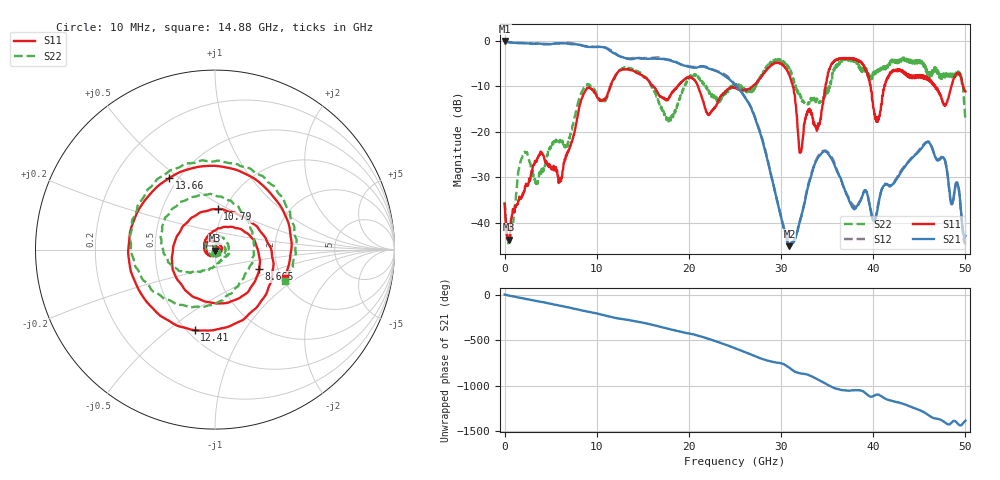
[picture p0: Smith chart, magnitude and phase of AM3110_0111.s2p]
# Hz S DB R 50.0
!freq dBS11 angS11 dBS21 angS21 dBS12 angS12 dBS22 angS22
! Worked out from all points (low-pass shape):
!   1601 points, 10 MHz to 50 GHz, reference 50 ohm
!   highest |S21| = -0.09 dB at 10 MHz (marker M1); lowest = -45.2 dB at 30.91 GHz (marker M2)
!   |S21| within 3 dB of the highest: start of sweep to 12.15 GHz
!   lowest |S11| = -43.8 dB at 478.7 MHz (marker M3), VSWR 1.01, Z = 50 - j0.647 ohm
!   |S11| at or under -10 dB: start of sweep to 11.47 GHz; 20.98 GHz to 26.95 GHz (5.968 GHz wide, 24.9 % of centre); 31.27 GHz to 34.83 GHz (3.558 GHz wide, 10.8 % of centre)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
!   |S22| runs from -44.6 to -3.8 dB; largest |S21 - S12| = 0.028
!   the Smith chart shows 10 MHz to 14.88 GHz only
!   S11 on the Smith chart (normalised r, x): 10 MHz: 1.01, -0.03; 8.665 GHz: 1.60, -0.37; 10.79 GHz: 0.93, +0.44; 12.41 GHz: 0.54, -0.62; 13.66 GHz: 0.45, +0.46; 14.88 GHz: 2.07, -0.78
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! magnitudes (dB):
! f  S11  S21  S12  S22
! 10 MHz  -35.9  -0.1  0.0  -35.4
! 478.7 MHz  -43.8  -0.4  -0.3  -44.6
! 1.978 GHz  -33.6  -0.6  -0.5  -25.2
! 6.103 GHz  -30.9  -0.6  -0.6  -22.2
! 8.352 GHz  -12.8  -1.1  -1.0  -11.4
! 8.665 GHz  -11.4  -1.2  -1.2  -10.4
! 10.79 GHz  -12.9  -1.5  -1.5  -13.2
! 12.41 GHz  -6.7  -3.4  -3.4  -6.7
! 13.66 GHz  -6.5  -4.1  -3.9  -6.2
! 14.88 GHz  -7.6  -4.0  -3.9  -7.3
! 16.69 GHz  -11.7  -4.0  -3.7  -13.4
! 25 GHz  -10.4  -9.7  -9.6  -9.9
! 30.91 GHz  -7.7  -45.2  -44.4  -6.4
! 32.1 GHz  -24.2  -39.3  -39.3  -12.1
! 33.35 GHz  -16.0  -29.1  -28.8  -12.7
! 35.94 GHz  -4.2  -28.1  -27.8  -5.5
! 38.85 GHz  -5.0  -34.0  -33.8  -6.1
! 40.44 GHz  -17.8  -37.5  -37.1  -6.5
! 41.69 GHz  -7.7  -31.8  -31.9  -5.8
! 46.03 GHz  -8.7  -22.4  -22.2  -6.9
! 49.16 GHz  -7.1  -31.5  -31.3  -7.5
! 50 GHz  -11.2  -42.9  -44.6  -17.6
